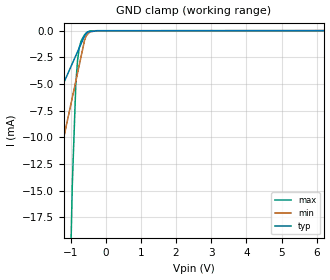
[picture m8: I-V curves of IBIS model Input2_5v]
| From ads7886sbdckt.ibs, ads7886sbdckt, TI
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[Model] Input2_5v
Model_type Input
Vinl = 800.000mV
Vinh = 4.60000V
C_comp 1.513pF 1.513pF 1.513pF
| variable typ   min   max
[Voltage Range] 5.00000V 4.75000V 5.25000V
[POWER Clamp Reference] 5.00000V 4.75000V 5.25000V
[GND Clamp Reference] 0.00000V 0.00000V 0.00000V
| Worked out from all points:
|   GND clamp passes 1 mA (typ) near -0.67 V on its own axis
[GND Clamp]
-5V       -33.15mA   -68.66mA   -619.5mA
-950mV    -3.079mA   -6.26mA    -14.4mA
-850mV    -2.336mA   -4.719mA   -4.96mA
-800mV    -1.965mA   -3.949mA   -2.742mA
-750mV    -1.593mA   -3.178mA   -1.559mA
-700mV    -1.222mA   -2.408mA   -957.5uA
-600mV    -479.4uA   -867.2uA   -374.1uA
-550mV    -258.7uA   -464.8uA   -183.6uA
-500mV    -115.6uA   -283.6uA   -101.3uA
-450mV    -94.32uA   -102.5uA   -18.94uA
-225mV    -9.14uA    -10.01uA   -1.333uA
10V       6.575uA    8.564uA    2.795uA
[POWER Clamp]
-5V       0A         0A         0A
10V       0A         0A         0A
